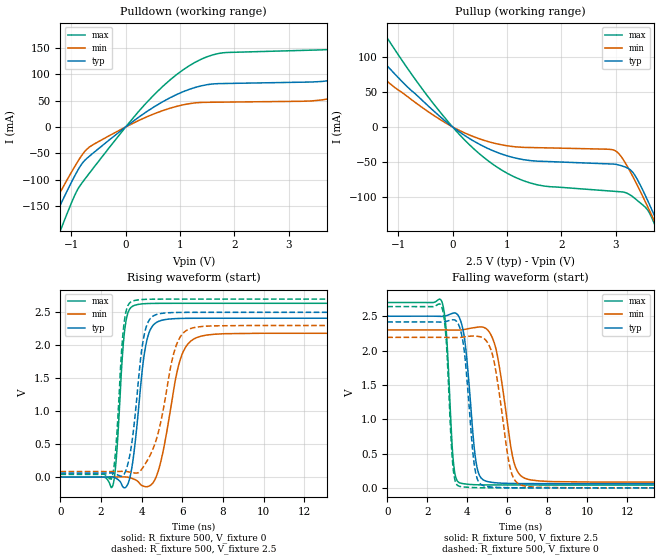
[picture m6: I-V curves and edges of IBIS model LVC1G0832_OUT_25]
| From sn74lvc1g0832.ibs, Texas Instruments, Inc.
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[Model]   LVC1G0832_OUT_25
Model_type  Output
Vref =   0
Rref =   500
Cref =   30p
Vmeas =   1.25
| variable   typ   min   max
C_comp   9.74pF   6.13pF   14.70pF
| C_pullup   9.53pF   6.13pF   11.20pF
| C_pulldown   9.95pF   6.62pF   14.70pF
[Temperature Range]   40   100   -40
| Ambient temperature   25   85   -40
[Voltage range]   2.5   2.3   2.7
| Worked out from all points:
|   slope of the pulldown table from 0 to 0.375 V, typ, clamps not added: 13.3 ohm
|   slope of the pullup table from 0 to 0.375 V, typ, clamps not added: 19 ohm
|   rising waveform, R_fixture 500, V_fixture 0: 20-80 % time 498ps typ, 780ps min, 315ps max; typ from 0 V to 2.41 V
|   falling waveform, R_fixture 500, V_fixture 2.5: 20-80 % time 431ps typ, 671ps min, 276ps max; typ from 2.5 V to 0.061 V
|   rising waveform, R_fixture 500, V_fixture 2.5: 20-80 % time 513ps typ, 887ps min, 317ps max; typ from 0.061 V to 2.5 V
|   falling waveform, R_fixture 500, V_fixture 0: 20-80 % time 416ps typ, 646ps min, 272ps max; typ from 2.42 V to 0 V
[Pulldown]
| LVC1G0832_OUT_25
|   Voltage   I(typ)   I(min)   I(max)
-5.5V     -1.06A     -941.4mA   -1.275A
-1.52V    -217.1mA   -184.1mA   -281.2mA
-1.26V    -160.6mA   -134.6mA   -212.3mA
-665mV    -55.38mA   -37.96mA   -87.52mA
385mV     28.96mA    19.04mA    46.35mA
1.275V    74.94mA    45.66mA    122.7mA
3.82V     89.61mA    55.07mA    148.2mA
5.34V     155.9mA    104.3mA    230.6mA
5.91V     186.3mA    52.55mA    280.7mA
6.525V    93.42mA    53.06mA    296.3mA
7.545V    94.06mA    54.02mA    161.3mA
11V       99.62mA    57.49mA    169.6mA
[Pullup]
| LVC1G0832_OUT_25
|   Voltage   I(typ)   I(min)   I(max)
-5.5V     533.4mA    418.6mA    746.4mA
-2.335V   192.2mA    147mA      274.9mA
-1.875V   147.9mA    112.2mA    212.9mA
-1.315V   97.38mA    72.9mA     141.5mA
-225mV    14.47mA    10.42mA    20.98mA
735mV     -33.88mA   -22.76mA   -53.28mA
1.56V     -49.18mA   -29.79mA   -83.17mA
2.98V     -53.48mA   -33.7mA    -92.52mA
3.325V    -66.27mA   -72.72mA   -100.9mA
3.755V    -135mA     -142.5mA   -147.1mA
3.835V    -149.5mA   -156.2mA   -162.8mA
11V       -1.609A    -1.492A    -1.841A
[Ramp]
| LVC1G0832_OUT_25
| variable   typ   min   max
dV/dt_r   1.54/5.34E-10   1.40/8.35E-10   1.68/3.40E-10
dV/dt_f   1.49/4.47E-10   1.36/6.91E-10   1.62/2.89E-10
R_load = 500
[Rising Waveform]
| LVC1G0832_OUT_25
R_fixture =   500
C_fixture =   0
L_fixture =   0
V_fixture =   0
V_fixture_min = 0
V_fixture_max = 0
|   Time   V(typ)   V(min)   V(max)
0s        125.3pV    6.247nV    2.314nV
2.565ns   2.075mV    -132.3uV   -140.1mV
2.75ns    -19.77mV   1.148mV    281.9mV
3.2ns     -158.5mV   2.301mV    2.313V
3.85ns    1.048V     -76.37mV   2.621V
4.165ns   1.934V     -143.7mV   2.631V
4.525ns   2.288V     -99.21mV   2.635V
5.96ns    2.407V     1.838V     2.636V
7.175ns   2.41V      2.154V     2.636V
50ns      2.41V      2.182V     2.636V
[Falling Waveform]
| LVC1G0832_OUT_25
R_fixture =   500
C_fixture =   0
L_fixture =   0
V_fixture =   2.5
V_fixture_min = 2.3
V_fixture_max = 2.7
|   Time   V(typ)   V(min)   V(max)
0s        2.5V       2.3V       2.7V
2.73ns    2.497V     2.3V       2.71V
2.955ns   2.508V     2.299V     2.257V
3.315ns   2.546V     2.297V     349.3mV
3.71ns    2.393V     2.3V       65.14mV
4.46ns    340.2mV    2.338V     45.11mV
5.12ns    85.44mV    2.261V     42.28mV
6.345ns   63.47mV    362.1mV    41.61mV
7.215ns   61.59mV    113.8mV    41.57mV
50ns      60.93mV    83.64mV    41.46mV
[Rising Waveform]
| LVC1G0832_OUT_25
R_fixture =   500
C_fixture =   0
L_fixture =   0
V_fixture =   2.5
V_fixture_min = 2.3
V_fixture_max = 2.7
|   Time   V(typ)   V(min)   V(max)
0s        60.91mV    83.6mV     41.45mV
2.515ns   64.09mV    83.45mV    -21.77mV
2.72ns    47.83mV    84.49mV    414.3mV
3.145ns   48.33mV    86.38mV    2.362V
3.72ns    1.072V     60.91mV    2.683V
4.035ns   2.001V     133.8mV    2.694V
4.38ns    2.386V     309.1mV    2.698V
5.705ns   2.498V     2.001V     2.7V
6.705ns   2.5V       2.276V     2.7V
50ns      2.5V       2.3V       2.7V
[Falling Waveform]
| LVC1G0832_OUT_25
R_fixture =   500
C_fixture =   0
L_fixture =   0
V_fixture =   0
V_fixture_min = 0
V_fixture_max = 0
|   Time   V(typ)   V(min)   V(max)
0s        2.416V     2.191V     2.64V
2.71ns    2.414V     2.192V     2.644V
2.945ns   2.423V     2.191V     2.152V
3.285ns   2.447V     2.189V     303.7mV
3.62ns    2.337V     2.191V     21.03mV
4.38ns    282.3mV    2.209V     3.195mV
4.93ns    22.79mV    2.149V     893.4uV
6.18ns    1.899mV    251mV      157.5uV
6.925ns   571.7uV    24mV       116.2uV
50ns      26.52uV    38.84uV    14.07uV
